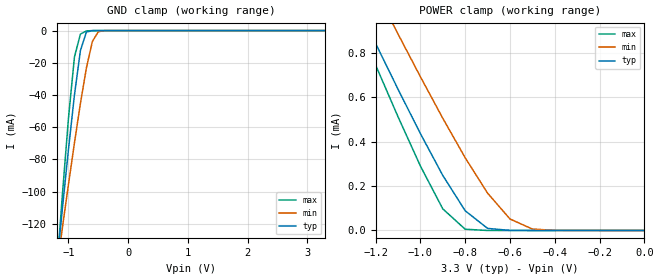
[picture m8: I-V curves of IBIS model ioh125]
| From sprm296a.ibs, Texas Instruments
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[Model]   ioh125
Model_type   Terminator
Polarity   Non-Inverting
| signals   Y
|   typ   min   max
C_comp   3.110p   3.034p   3.113p
|   typ   min   max
[Temperature Range]   25   -40   125
|   typ   min   max
[Voltage Range]   3.30V   3.00V   3.60V
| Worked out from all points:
|   GND clamp passes 1 mA (typ) near -0.70 V on its own axis
|   POWER clamp passes 1 mA (typ) near -1.28 V on its own axis
[GND_clamp]
|   Voltage   I(typ)   I(min)   I(max)
-3.3V     -988mA     -752.6mA   -1.27A
-1.2V     -147.1mA   -149mA     -150.5mA
-1.1V     -109.8mA   -122mA     -101mA
-1V       -73.75mA   -95.47mA   -54.42mA
-900mV    -40.03mA   -69.74mA   -16.37mA
-800mV    -12.4mA    -45.28mA   -2.185mA
-700mV    -937.4uA   -23.22mA   -216.5uA
-600mV    -39.35uA   -6.774mA   -12.38uA
-500mV    -1.944uA   -693.2uA   -432.6nA
-400mV    -88.95nA   -41.39uA   -11.11nA
3.3V      177.6pA    27.49nA    177.6pA
[POWER_clamp]
|   Voltage   I(typ)   I(min)   I(max)
-3.3V     5.414mA    5.399mA    5.945mA
-1.3V     1.052mA    1.28mA     983.4uA
-1.2V     842.7uA    1.081mA    745.4uA
-1.1V     636.6uA    885.2uA    512.6uA
-1V       436.5uA    692.6uA    290.3uA
-900mV    247.9uA    505.4uA    97.32uA
-800mV    88.8uA     327.5uA    5.525uA
-700mV    9.316uA    168.2uA    52.05nA
-600mV    265nA      51.74uA    977pA
-500mV    6.484nA    6.448uA    444.1pA
-400mV    399.7pA    429.5nA    355.3pA
0V        1pA        1pA        1pA
